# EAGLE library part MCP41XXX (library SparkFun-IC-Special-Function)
Digital Potentiometer - 10K SPI controlled single digital potentiometer by Microchip Datasheet SparkFun Products Storefront component: Digital Potentiometer - 10K (COM-10613)
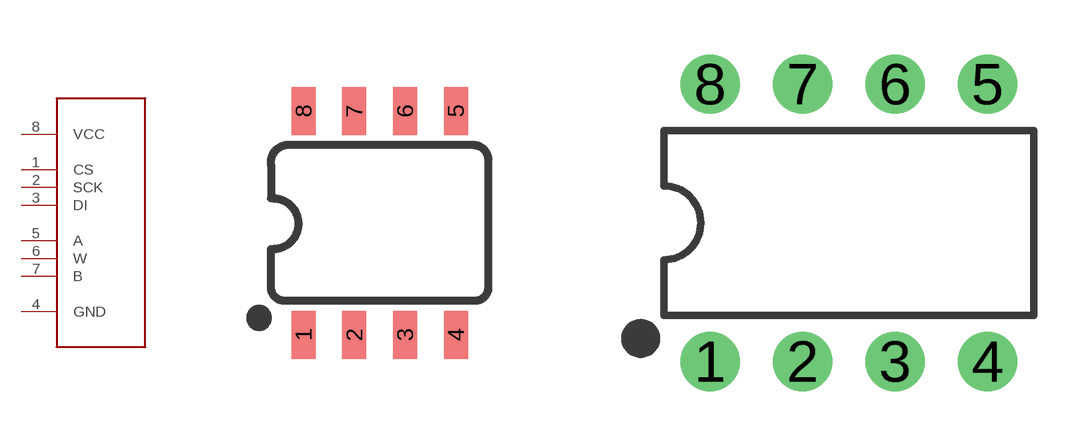
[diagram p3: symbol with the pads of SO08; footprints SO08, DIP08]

Designator prefix U

## MCP41XXX (PROD_ID: NA-XXXXX; VALUE: MCP41XXX)  [SO08]
1  CS
2  SCK
3  DI
4  GND
5  A
6  W
7  B
8  VCC

## MCP41XXXDIL (PROD_ID: RES-13155; VALUE: MCP41XXX)  [DIP08]
Pads as for SO08

## Footprint SO08 (pad centres in mm)
SOIC, 0.15 inch width
smd 0.6 x 1.2: 1 -1.905,-2.8; 2 -0.635,-2.8; 3 0.635,-2.8; 4 1.905,-2.8; 5 1.905,2.8; 6 0.635,2.8; 7 -0.635,2.8; 8 -1.905,2.8

## Footprint DIP08 (pad centres in mm)
Dual In Line Package
drill 0.813 pad 1.626: 1 -3.81,-3.81; 2 -1.27,-3.81; 3 1.27,-3.81; 4 3.81,-3.81; 5 3.81,3.81; 6 1.27,3.81; 7 -1.27,3.81; 8 -3.81,3.81

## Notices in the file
Licensing: Creative Commons ShareAlike 4.0 International - https://creativecommons.org/licenses/by-sa/4.0
